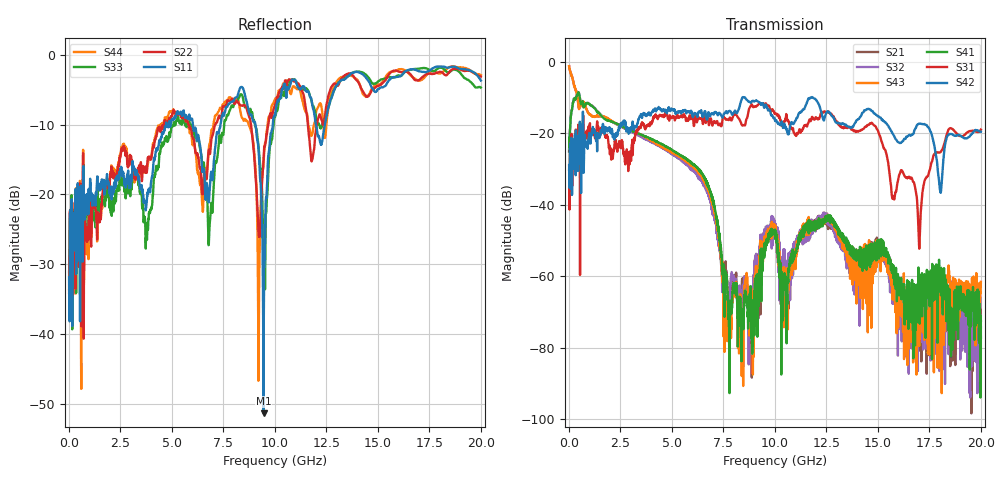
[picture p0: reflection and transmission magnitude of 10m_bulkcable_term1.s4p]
# MHz S MA R 50.00
! FREQ  S11  S12  S13  S14
!  S21  S22  S23  S24
!  S31  S32  S33  S34
!  S41  S42  S43  S44
!  MAG  ANG  MAG  ANG  MAG  ANG  MAG  ANG
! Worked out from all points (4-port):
!   2000 points, 10 MHz to 20 GHz, reference 50 ohm
!   strongest paths, dB at 10 MHz, 5.01 GHz, 10.01 GHz, 15.01 GHz, 20 GHz:
!     S42: -30.2, -13.2, -16.4, -15.1, -19.5
!     S31: -28.9, -15.3, -14.2, -19.3, -18.9
!     S41: -25.0, -24.6, -46.9, -51.5, -77.3
!     S43: -1.1, -25.2, -48.5, -56.1, -61.6
!     S32: -25.0, -25.9, -45.4, -52.9, -74.3
!     S21: -1.1, -25.1, -47.5, -53.4, -72.4
!   lowest |S11| = -51.4 dB at 9.45 GHz (marker M1), VSWR 1.01, Z = 50.1 - j0.263 ohm
!   |S11| at or under -10 dB: start of sweep to 4.714 GHz; 6.022 GHz to 7.359 GHz (1.337 GHz wide, 20 % of centre); 9.056 GHz to 9.899 GHz (842.8 MHz wide, 8.89 % of centre)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
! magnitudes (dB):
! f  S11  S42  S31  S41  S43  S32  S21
! 10 MHz  -31.9  -30.2  -28.9  -25.0  -1.1  -25.0  -1.1
! 6.28 GHz  -11.6  -14.1  -15.6  -29.8  -31.0  -31.5  -31.3
! 7.77 GHz  -7.0  -13.7  -16.2  -72.3  -69.7  -73.9  -72.3
! 9.45 GHz  -51.4  -12.1  -11.7  -53.4  -51.1  -50.6  -51.2
! 10.41 GHz  -4.6  -18.2  -17.0  -63.4  -64.3  -52.5  -64.8
! 17.01 GHz  -2.4  -17.2  -52.3  -67.8  -66.9  -66.2  -64.5
! 20 GHz  -3.7  -19.5  -18.9  -77.3  -61.6  -74.3  -72.4
